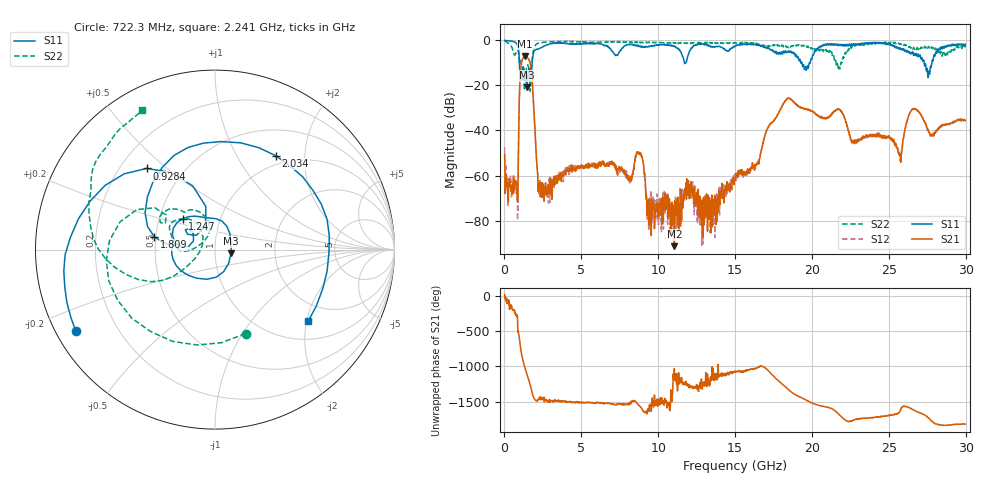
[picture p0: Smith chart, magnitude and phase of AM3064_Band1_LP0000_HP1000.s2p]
# Hz S DB R 50.0
!freq dBS11 angS11 dBS21 angS21 dBS12 angS12 dBS22 angS22
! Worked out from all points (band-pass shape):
!   1600 points, 10 MHz to 29.98 GHz, reference 50 ohm
!   highest |S21| = -6.94 dB at 1.341 GHz (marker M1); lowest = -91.4 dB at 11.05 GHz (marker M2)
!   |S21| within 3 dB of the highest: 1.105 GHz to 1.666 GHz (561.6 MHz wide, 40.5 % of centre)
!   lowest |S11| = -20.7 dB at 1.453 GHz (marker M3), VSWR 1.20, Z = 59.8 - j2.39 ohm
!   |S11| at or under -10 dB: 973.4 MHz to 1.799 GHz (825.9 MHz wide, 59.6 % of centre); 19.35 GHz to 19.83 GHz (470.9 MHz wide, 2.4 % of centre); 27.3 GHz to 27.79 GHz (497.2 MHz wide, 1.8 % of centre)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
!   |S22| runs from -22.6 to -0.2 dB; largest |S21 - S12| = 0.0052
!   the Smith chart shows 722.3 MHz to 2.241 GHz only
!   S11 on the Smith chart (normalised r, x): 722.3 MHz: 0.06, -0.27; 928.4 MHz: 0.31, +0.43; 1.247 GHz: 0.66, +0.24; 1.809 GHz: 0.49, +0.08; 2.034 GHz: 0.86, +1.47; 2.241 GHz: 1.47, -2.04
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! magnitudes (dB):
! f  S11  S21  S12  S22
! 10 MHz  0.0  -50.5  -47.4  -0.2
! 722.3 MHz  -0.9  -62.3  -63.5  -6.1
! 928.4 MHz  -4.6  -39.9  -39.8  -6.2
! 1.247 GHz  -12.1  -7.4  -7.4  -16.1
! 1.341 GHz  -15.0  -6.9  -6.9  -17.5
! 1.453 GHz  -20.7  -7.2  -7.1  -11.8
! 1.809 GHz  -9.2  -18.4  -18.3  -8.0
! 2.034 GHz  -4.1  -46.2  -46.0  -1.9
! 2.241 GHz  -3.7  -65.0  -67.9  -1.2
! 5.015 GHz  -1.5  -55.3  -55.9  -0.7
! 8.126 GHz  -1.8  -61.5  -63.9  -0.8
! 8.745 GHz  -2.7  -50.3  -50.3  -1.2
! 9.344 GHz  -2.9  -73.9  -77.5  -1.0
! 10 GHz  -2.0  -78.2  -74.1  -0.9
! 11.05 GHz  -2.4  -91.4  -77.4  -1.2
! 15 GHz  -2.6  -62.1  -61.2  -1.2
! 18.34 GHz  -5.4  -26.2  -26.0  -2.6
! 19.99 GHz  -8.3  -31.3  -31.3  -3.4
! 25 GHz  -1.4  -42.6  -42.7  -1.1
! 26.63 GHz  -6.8  -30.2  -30.3  -3.2
! 27.56 GHz  -16.5  -40.1  -40.0  -2.7
! 29.98 GHz  -1.7  -35.6  -35.5  -3.1
